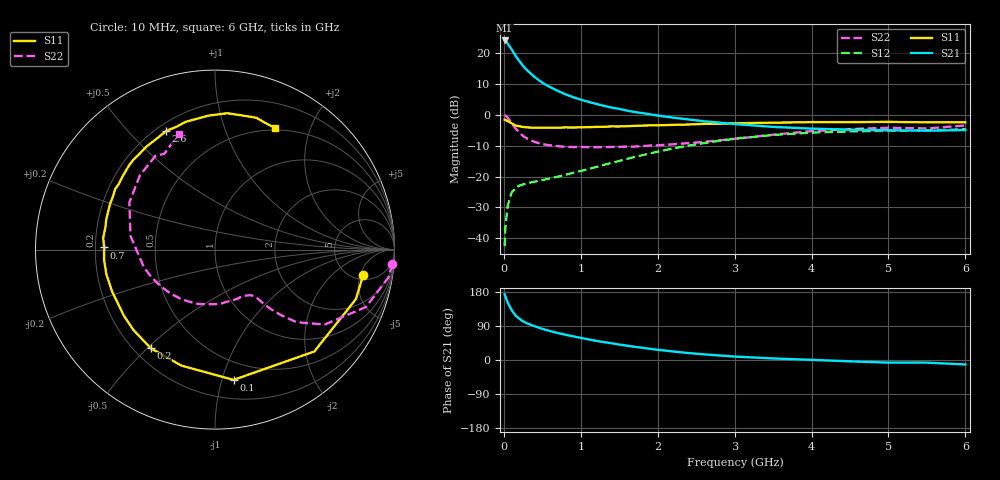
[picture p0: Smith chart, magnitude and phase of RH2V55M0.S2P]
! SIEMENS Small Signal Semiconductors
! BFR106
! Si NPN RF Bipolar Junction Transistor in SOT23
! VCE = 2.5 V  IC = 5 mA
! Common Emitter S-Parameters:  August  1996
# GHz  S  MA  R  50
!  f  S11  S21  S12  S22
! GHz  MAG  ANG  MAG  ANG  MAG  ANG  MAG  ANG
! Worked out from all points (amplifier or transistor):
!   36 points, 10 MHz to 6 GHz, reference 50 ohm
!   highest |S21| = 24.2 dB at 10 MHz (marker M1)
!   |S21| within 3 dB of that: start of sweep to 104.3 MHz
!   unconditionally stable (mu >= 1): 618.6 MHz to 2.122 GHz; 4.322 GHz to end of sweep
!   at 250 MHz: K = 0.51, MSG = 19.2 dB, |S12| = -22.6 dB
!   at 1.4 GHz: K = 1.15, MAG = 6.6 dB, |S12| = -15.6 dB
!   at 6 GHz: K = 1.02, MAG = -1.1 dB, |S12| = -4.7 dB
!   S11 on the Smith chart (normalised r, x): 10 MHz: 5.93, -5.62; 100 MHz: 0.35, -1.09; 200 MHz: 0.27, -0.51; 700 MHz: 0.24, +0.01; 2.6 GHz: 0.24, +0.64; 6 GHz: 0.48, +1.51
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0.01  0.838 -9.7  16.15 173.4  0.0074 87.0  0.9909 -4.6
0.02  0.8321 -19.4  15.91 168.2  0.0148 80.9  0.9791 -9.1
0.05  0.7928 -45.7  14.42 151.7  0.0335 66.7  0.8998 -20.8
0.1  0.7332 -81.9  11.67 132.1  0.0545 52.4  0.7405 -34.3
0.15  0.6729 -106.2  9.192 118.0  0.0649 43.3  0.608 -41.7
0.2  0.656 -123.1  7.52 109.2  0.0711 39.1  0.5209 -44.7
0.25  0.6378 -135.7  6.247 102.0  0.0745 36.6  0.4547 -46.8
0.3  0.627 -144.3  5.333 97.0  0.0775 36.8  0.4154 -47.9
0.4  0.6188 -157.9  4.122 89.0  0.0824 37.4  0.3633 -48.9
0.5  0.6207 -167.1  3.337 82.2  0.0874 39.5  0.3359 -50.1
0.6  0.6205 -174.8  2.83 76.4  0.0934 42.1  0.3205 -52.4
0.7  0.618 178.9  2.46 71.3  0.0992 45.2  0.3112 -55.3
0.9  0.6229 168.9  1.939 62.4  0.1146 50.1  0.3007 -61.2
1.1  0.6325 159.8  1.629 54.4  0.1322 54.3  0.2995 -69.5
1.3  0.6409 152.4  1.404 47.3  0.1548 56.9  0.2985 -78.1
1.6  0.656 141.9  1.175 37.8  0.1931 58.5  0.3049 -92.5
2.2  0.6892 123.8  0.902 22.5  0.285 54.8  0.3336 -123.8
2.6  0.7148 112.3  0.788 15.0  0.3483 49.1  0.3643 -145.8
3.5  0.747 92.9  0.639 4.1  0.4726 32.4  0.4769 170.8
4.5  0.763 78.1  0.575 -3.5  0.5384 13.8  0.5882 135.3
5.5  0.7579 67.4  0.554 -7.0  0.5609 2.7  0.6039 117.9
6  0.7556 63.6  0.568 -11.8  0.5852 -4.8  0.6734 107.5
